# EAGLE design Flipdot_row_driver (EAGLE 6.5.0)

## Sheet 1 of 2: Flip dot driver
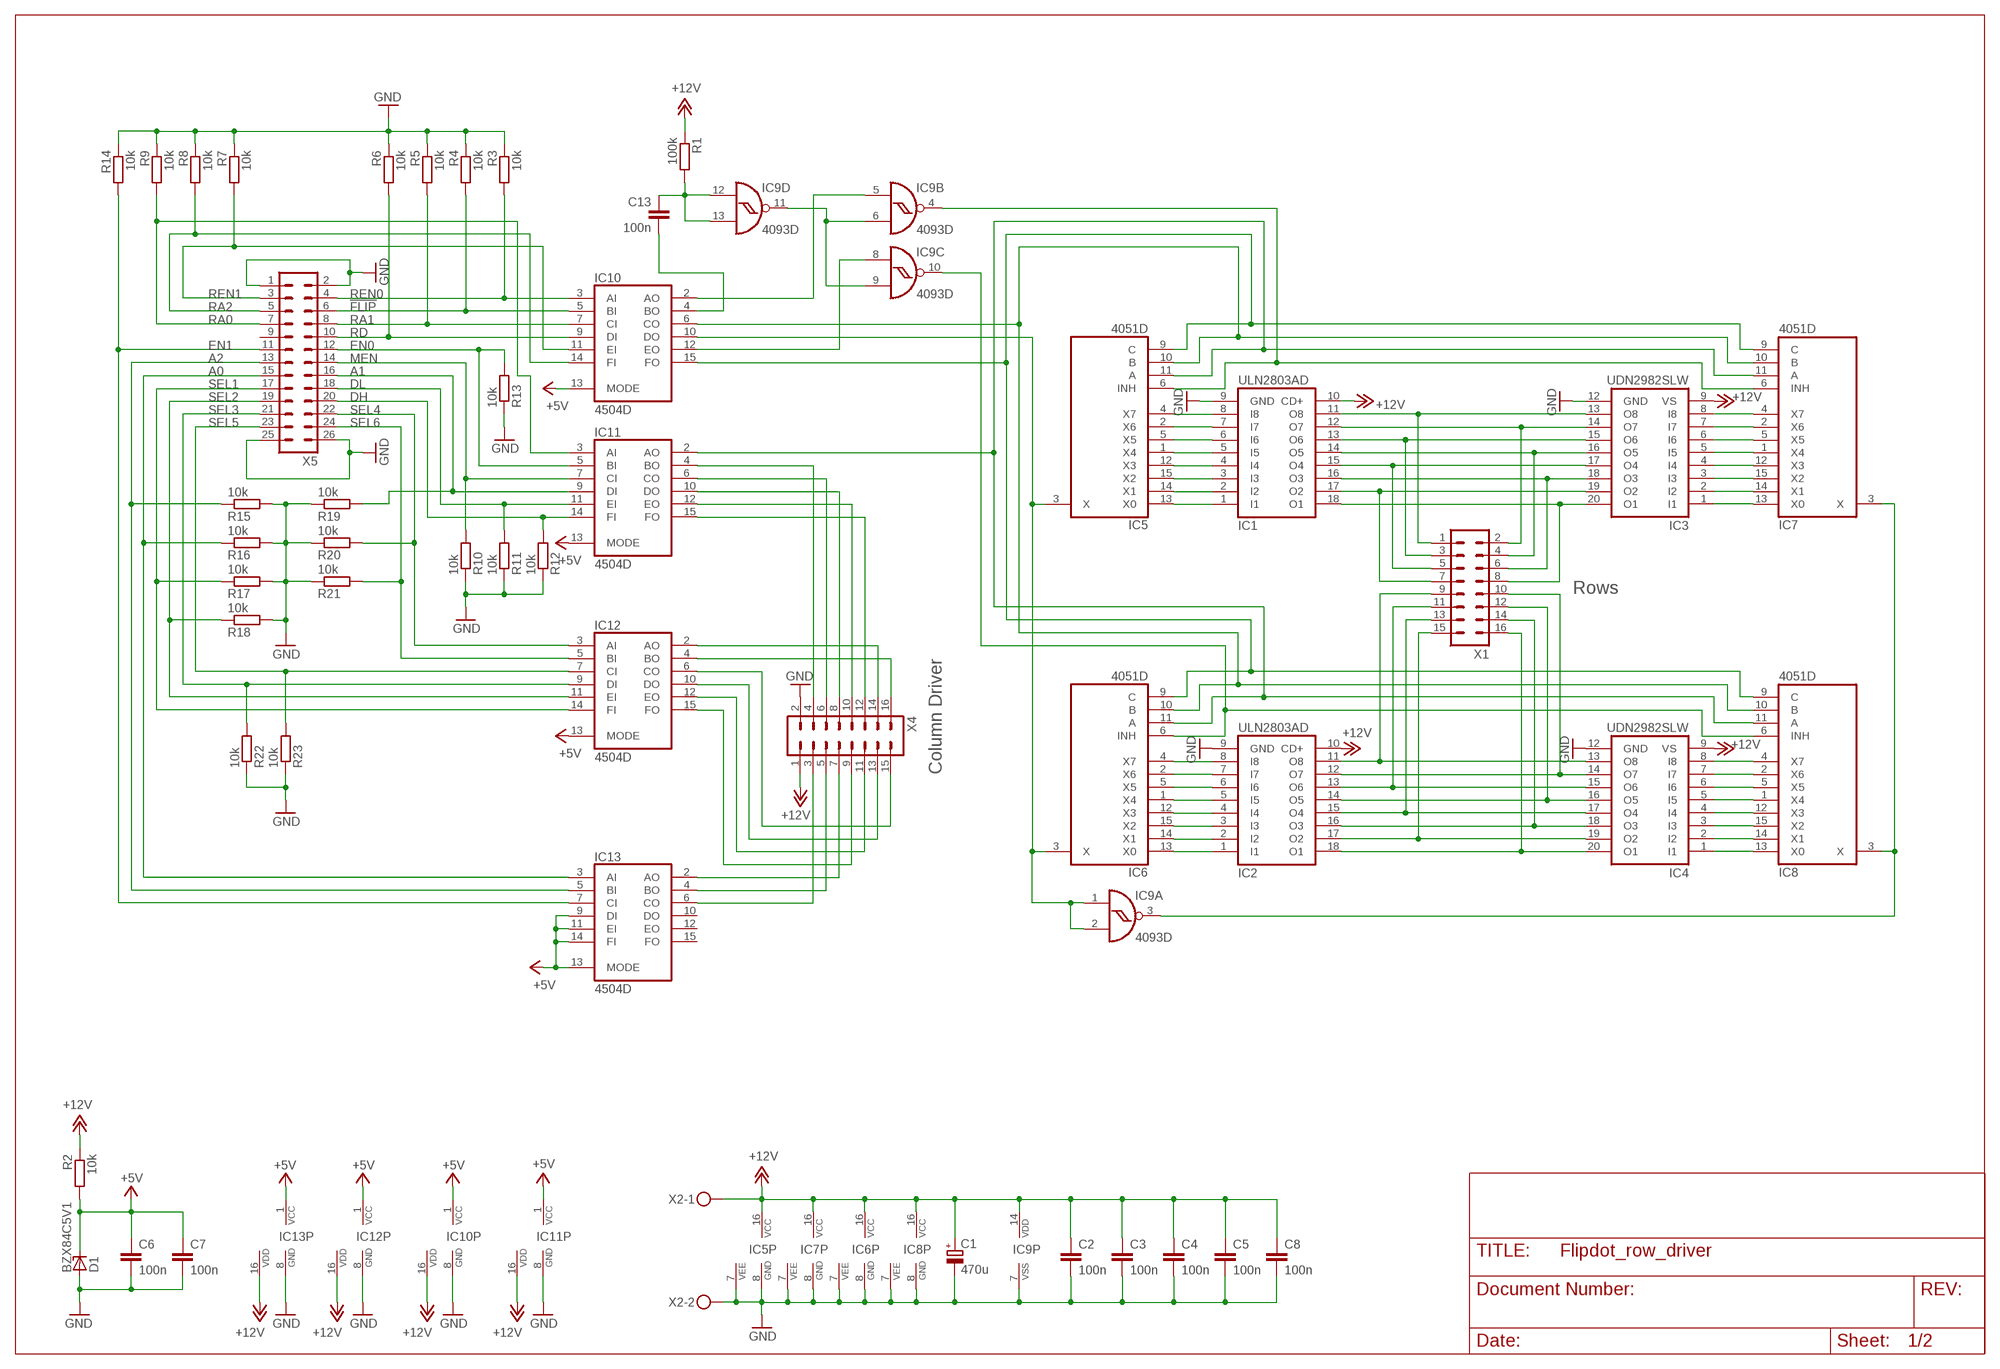
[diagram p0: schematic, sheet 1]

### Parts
C1  470u  CPOL-EUE3.5-8  [E3,5-8]
C2  100n  C-EUC0603K  [C0603K]
C3  100n  C-EUC0603K  [C0603K]
C4  100n  C-EUC0603K  [C0603K]
C5  100n  C-EUC0603K  [C0603K]
C6  100n  C-EUC0603K  [C0603K]
C7  100n  C-EUC0603K  [C0603K]
C8  100n  C-EUC0603K  [C0603K]
C13  100n  C-EUC0603K  [C0603K]
D1  BZX84C5V1  BZX84CSMD  [TO236]
IC1  ULN2803AD  [SO18W]
IC2  ULN2803AD  [SO18W]
IC3  UDN2982SLW  UDN2984SLW  [SO20W]
IC4  UDN2982SLW  UDN2984SLW  [SO20W]
IC5  4051D  [SO16]
IC6  4051D  [SO16]
IC7  4051D  [SO16]
IC8  4051D  [SO16]
IC9  4093D  [SO14]
IC10  4504D  [SO16]
IC11  4504D  [SO16]
IC12  4504D  [SO16]
IC13  4504D  [SO16]
R1  100k  R-EU_R0603  [R0603]
R2  10k  R-EU_R0603  [R0603]
R3  10k  R-EU_R0603  [R0603]
R4  10k  R-EU_R0603  [R0603]
R5  10k  R-EU_R0603  [R0603]
R6  10k  R-EU_R0603  [R0603]
R7  10k  R-EU_R0603  [R0603]
R8  10k  R-EU_R0603  [R0603]
R9  10k  R-EU_R0603  [R0603]
R10  10k  R-EU_R0603  [R0603]
R11  10k  R-EU_R0603  [R0603]
R12  10k  R-EU_R0603  [R0603]
R13  10k  R-EU_R0603  [R0603]
R14  10k  R-EU_R0603  [R0603]
R15  10k  R-EU_R0603  [R0603]
R16  10k  R-EU_R0603  [R0603]
R17  10k  R-EU_R0603  [R0603]
R18  10k  R-EU_R0603  [R0603]
R19  10k  R-EU_R0603  [R0603]
R20  10k  R-EU_R0603  [R0603]
R21  10k  R-EU_R0603  [R0603]
R22  10k  R-EU_R0603  [R0603]
R23  10k  R-EU_R0603  [R0603]
X1  ML16  [ML16]
X2  MKDSN1,5/2-5,08  [MKDSN1,5/2-5,08]
X4  ML16  [ML16]
X5  ML26  [ML26]

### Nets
!FLIP: IC10.5(BI) R4.2 X5.6
+5V: C6.1 C7.1 D1.C IC10.1(VCC) IC10.13(MODE) IC11.1(VCC) IC11.13(MODE) IC12.1(VCC) IC12.13(MODE) IC13.1(VCC) IC13.9(DI) IC13.11(EI) IC13.13(MODE) IC13.14(FI) R2.2
+12V: C1.+ C2.1 C3.1 C4.1 C5.1 C8.1 IC1.10(CD+) IC2.10(CD+) IC3.9(VS) IC4.9(VS) IC5.16(VCC) IC6.16(VCC) IC7.16(VCC) IC8.16(VCC) IC9.14(P:VDD) IC10.16(VDD) IC11.16(VDD) IC12.16(VDD) IC13.16(VDD) R1.1 R2.1 X2.1 X4.1 ; also sheet 2
A0: IC13.3(AI) R16.1 X5.15
A1: IC11.9(DI) R19.2 X5.16
A2: IC13.5(BI) R15.1 X5.13
DH: IC11.14(FI) R12.2 X5.20
DL: IC11.11(EI) R11.2 X5.18
EN0: IC11.5(BI) R13.2 X5.12
EN1: IC13.7(CI) R14.2 X5.11
GND: C1.- C2.2 C3.2 C4.2 C5.2 C6.2 C7.2 C8.2 D1.A IC1.9(GND) IC2.9(GND) IC3.12(GND) IC4.12(GND) IC5.7(VEE) IC5.8(GND) IC6.7(VEE) IC6.8(GND) IC7.7(VEE) IC7.8(GND) IC8.7(VEE) IC8.8(GND) IC9.7(P:VSS) IC10.8(GND) IC11.8(GND) IC12.8(GND) IC13.8(GND) R3.1 R4.1 R5.1 R6.1 R7.1 R8.1 R9.1 R10.1 R11.1 R12.1 R13.1 R14.1 R15.2 R16.2 R17.2 R18.2 R19.1 R20.1 R21.1 R22.1 R23.1 X2.2 X4.2 X5.1 X5.2 X5.25 X5.26 ; also sheet 2
MEN: IC11.7(CI) R10.2 X5.14
N$1: IC11.4(BO) X4.4
N$2: IC1.12(O7) IC3.14(O7) X1.2
N$3: IC11.6(CO) X4.6
N$4: IC1.14(O5) IC3.16(O5) X1.4
N$5: IC11.10(DO) X4.8
N$6: IC1.16(O3) IC3.18(O3) X1.6
N$7: IC11.12(EO) X4.10
N$8: IC1.18(O1) IC3.20(O1) X1.8
N$9: IC11.15(FO) X4.12
N$10: IC1.11(O8) IC3.13(O8) X1.1
N$11: IC12.2(AO) X4.14
N$12: IC1.13(O6) IC3.15(O6) X1.3
N$13: IC12.4(BO) X4.16
N$14: IC1.15(O4) IC3.17(O4) X1.5
N$15: IC13.6(CO) X4.3
N$16: IC1.17(O2) IC3.19(O2) X1.7
N$17: IC1.8(I8) IC5.4(X7)
N$18: IC1.7(I7) IC5.2(X6)
N$19: IC1.6(I6) IC5.5(X5)
N$20: IC1.5(I5) IC5.1(X4)
N$21: IC1.4(I4) IC5.12(X3)
N$22: IC1.3(I3) IC5.15(X2)
N$23: IC1.2(I2) IC5.14(X1)
N$24: IC1.1(I1) IC5.13(X0)
N$25: IC3.5(I5) IC7.1(X4)
N$26: IC3.7(I7) IC7.2(X6)
N$27: IC3.8(I8) IC7.4(X7)
N$28: IC3.6(I6) IC7.5(X5)
N$29: IC3.4(I4) IC7.12(X3)
N$30: IC3.1(I1) IC7.13(X0)
N$31: IC3.2(I2) IC7.14(X1)
N$32: IC3.3(I3) IC7.15(X2)
N$33: IC13.4(BO) X4.5
N$34: IC13.2(AO) X4.7
N$35: IC6.6(INH) IC8.6(INH) IC9.10(C:O)
N$36: C13.1 IC9.12(D:I0) IC9.13(D:I1) R1.2
N$37: IC12.15(FO) X4.9
N$38: IC12.12(EO) X4.11
N$39: IC9.6(B:I1) IC9.9(C:I1) IC9.11(D:O)
N$40: IC12.10(DO) X4.13
N$41: IC12.6(CO) X4.15
N$43: IC5.3(X) IC6.3(X) IC9.1(A:I0) IC9.2(A:I1) IC10.10(DO)
N$46: IC2.12(O7) IC4.14(O7) X1.10
N$48: IC2.14(O5) IC4.16(O5) X1.12
N$50: IC2.16(O3) IC4.18(O3) X1.14
N$52: IC2.18(O1) IC4.20(O1) X1.16
N$54: IC2.11(O8) IC4.13(O8) X1.9
N$56: IC2.13(O6) IC4.15(O6) X1.11
N$58: IC2.15(O4) IC4.17(O4) X1.13
N$60: IC2.17(O2) IC4.19(O2) X1.15
N$61: IC2.8(I8) IC6.4(X7)
N$62: IC2.7(I7) IC6.2(X6)
N$63: IC2.6(I6) IC6.5(X5)
N$64: IC2.5(I5) IC6.1(X4)
N$65: IC2.4(I4) IC6.12(X3)
N$66: IC2.3(I3) IC6.15(X2)
N$67: IC2.2(I2) IC6.14(X1)
N$68: IC2.1(I1) IC6.13(X0)
N$69: IC4.5(I5) IC8.1(X4)
N$70: IC4.7(I7) IC8.2(X6)
N$71: IC4.8(I8) IC8.4(X7)
N$72: IC4.6(I6) IC8.5(X5)
N$73: IC4.4(I4) IC8.12(X3)
N$74: IC4.1(I1) IC8.13(X0)
N$75: IC4.2(I2) IC8.14(X1)
N$76: IC4.3(I3) IC8.15(X2)
N$77: IC5.6(INH) IC7.6(INH) IC9.4(B:O)
N$100: IC9.5(B:I0) IC10.2(AO)
N$101: C13.2 IC10.4(BO)
N$102: IC5.10(B) IC6.10(B) IC7.10(B) IC8.10(B) IC10.6(CO)
N$104: IC9.8(C:I0) IC10.12(EO)
N$105: IC5.9(C) IC6.9(C) IC7.9(C) IC8.9(C) IC10.15(FO)
N$106: IC5.11(A) IC6.11(A) IC7.11(A) IC8.11(A) IC11.2(AO)
N$110: IC7.3(X) IC8.3(X) IC9.3(A:O)
RA0: IC11.3(AI) R9.2 X5.7
RA1: IC10.7(CI) R5.2 X5.8
RA2: IC10.14(FI) R8.2 X5.5
RD: IC10.9(DI) R6.2 X5.10
REN0: IC10.3(AI) R3.2 X5.4
REN1: IC10.11(EI) R7.2 X5.3
SEL1: IC12.14(FI) R17.1 X5.17
SEL2: IC12.11(EI) R18.1 X5.19
SEL3: IC12.9(DI) R22.2 X5.21
SEL4: IC12.3(AI) R20.2 X5.22
SEL5: IC12.7(CI) R23.2 X5.23
SEL6: IC12.5(BI) R21.2 X5.24
Unconnected: IC13.10(DO) IC13.12(EO) IC13.15(FO) X5.9

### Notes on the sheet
- Rows
- Column Driver

## Sheet 2 of 2: Flip dot master
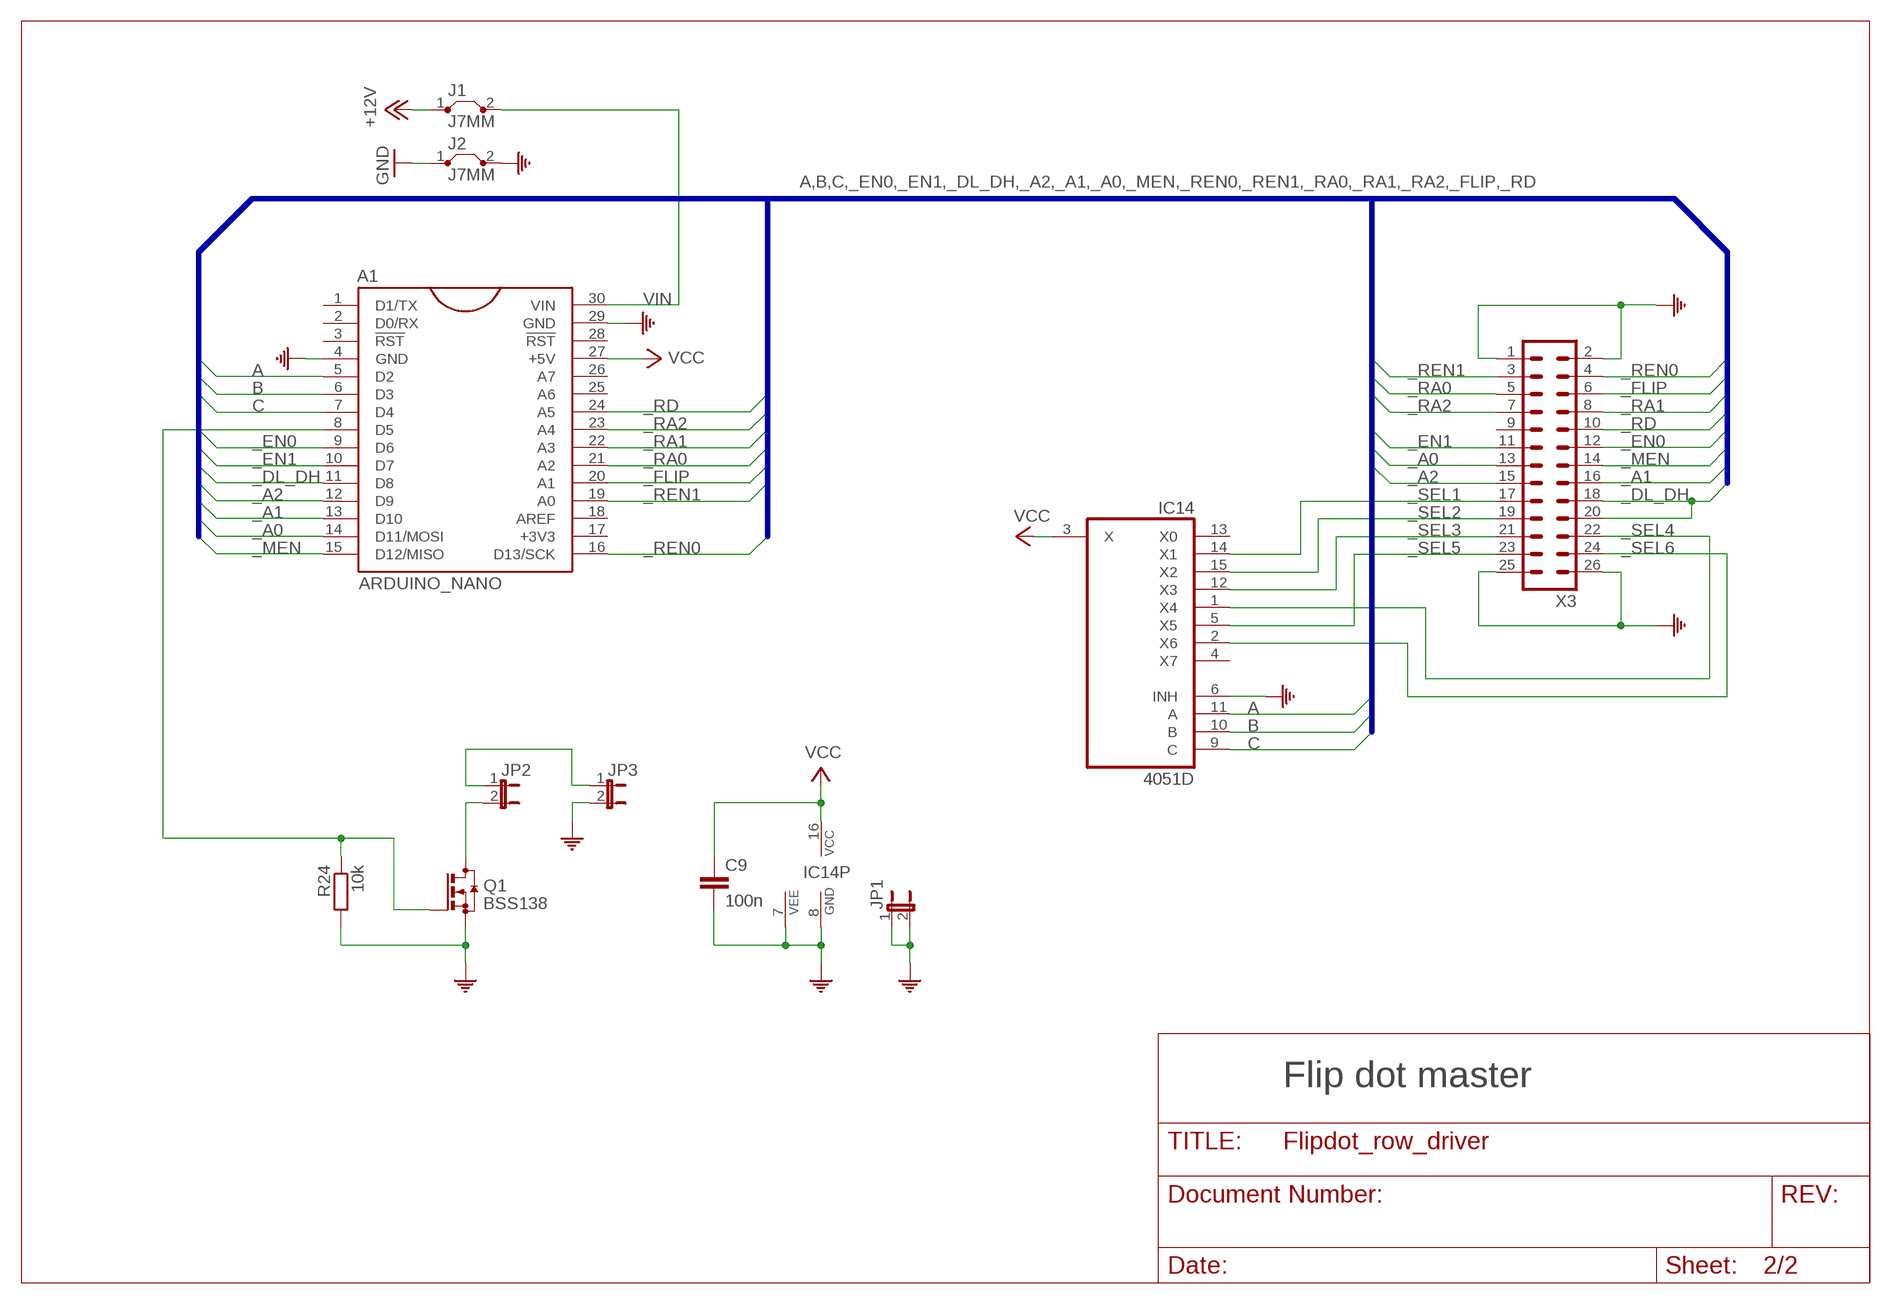
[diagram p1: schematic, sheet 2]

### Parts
A1  ARDUINO_NANO  [ARDUINO_NANO]
C9  100n  C-EUC0603K  [C0603K]
IC14  4051D  [SO16]
J1  J7MM  [07]
J2  J7MM  [07]
JP1  JP1E  [JP1]
JP2  JP1E  [JP1]
JP3  JP1E  [JP1]
Q1  BSS138  BSS123  [SOT23]
R24  10k  R-EU_R0603  [R0603]
X3  ML26  [ML26]

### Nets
+12V: J1.1 ; also sheet 1
_A0: A1.14(D11/MOSI) X3.13
_A1: A1.13(D10) X3.16
_A2: A1.12(D9) X3.15
_DL_DH: A1.11(D8) X3.18 X3.20
_EN0: A1.9(D6) X3.12
_EN1: A1.10(D7) X3.11
_FLIP: A1.20(A1) X3.6
_MEN: A1.15(D12/MISO) X3.14
_RA0: A1.21(A2) X3.5
_RA1: A1.22(A3) X3.8
_RA2: A1.23(A4) X3.7
_RD: A1.24(A5) X3.10
_REN0: A1.16(D13/SCK) X3.4
_REN1: A1.19(A0) X3.3
_SEL1: IC14.14(X1) X3.17
_SEL2: IC14.15(X2) X3.19
_SEL3: IC14.12(X3) X3.21
_SEL4: IC14.1(X4) X3.22
_SEL5: IC14.5(X5) X3.23
_SEL6: IC14.2(X6) X3.24
A: A1.5(D2) IC14.11(A)
B: A1.6(D3) IC14.10(B)
C: A1.7(D4) IC14.9(C)
COM: A1.4(GND) A1.29(GND) C9.2 IC14.6(INH) IC14.7(VEE) IC14.8(GND) J2.2 JP1.1 JP1.2 JP3.2 Q1.2(S) R24.2 X3.1 X3.2 X3.25 X3.26
GND: J2.1 ; also sheet 1
N$42: A1.8(D5) Q1.1(G) R24.1
N$44: JP2.2 Q1.3(D)
N$45: JP2.1 JP3.1
VCC: A1.27(+5V) C9.1 IC14.3(X) IC14.16(VCC)
VIN: A1.30(VIN) J1.2
Unconnected: A1.1(D1/TX) A1.2(D0/RX) A1.3(!RST) A1.17(+3V3) A1.18(AREF) A1.25(A6) A1.26(A7) A1.28(!RST) IC14.4(X7) IC14.13(X0) X3.9

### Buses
A,B,C,_EN0,_EN1,_DL_DH,_A2,_A1,_A0,_MEN,_REN0,_REN1,_RA0,_RA1,_RA2,_FLIP,_RD

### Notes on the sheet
- Flip dot master

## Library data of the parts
A1 = Brunner:ARDUINO_NANO: Arduino Nano plug in module
C1 = rcl:CPOL-EU: POLARIZED CAPACITOR, European symbol
C2-C9 C13 = rcl:C-EU: CAPACITOR, European symbol
D1 = diode:BZX84CSMD: Z DIODE
IC1 IC2 = Brunner:ULN2803A: DRIVER ARRAY
IC3 IC4 = uln-udn:UDN298*: DRIVER ARRAY Source: Allegro Microsystems Inc. / UDN2981-UDN2984.pdf
IC5-IC8 IC14 = 40xx:4051: 8-channel ANALOG MULTIPLEXER
IC9 = 40xx:4093: Quad 2-input NAND schmitt trigger
IC10-IC13 = 45xx:4504: TTL or CMOS to CMOS hex LEVEL SHIFTER
J1 J2 = jumper:J: Bridge
JP1-JP3 = jumper:JP1E: JUMPER
Q1 = transistor-small-signal:BSS123: N-CHANNEL MOS FET
R1-R24 = rcl:R-EU_: RESISTOR, European symbol
X1 X4 = con-ml:ML16: HARTING; OC_FARNELL: unknown; OC_NEWARK: unknown
X2 = con-phoenix-508:MKDSN1,5/2-5,08: MKDSN 1,5/ 2-5,08 Printklemme; MPN: MKDSN 1,5/2-5.08; OC_FARNELL: 1792903; OC_NEWARK: 30M2397
X3 X5 = con-ml:ML26: HARTING; OC_FARNELL: unknown; OC_NEWARK: unknown

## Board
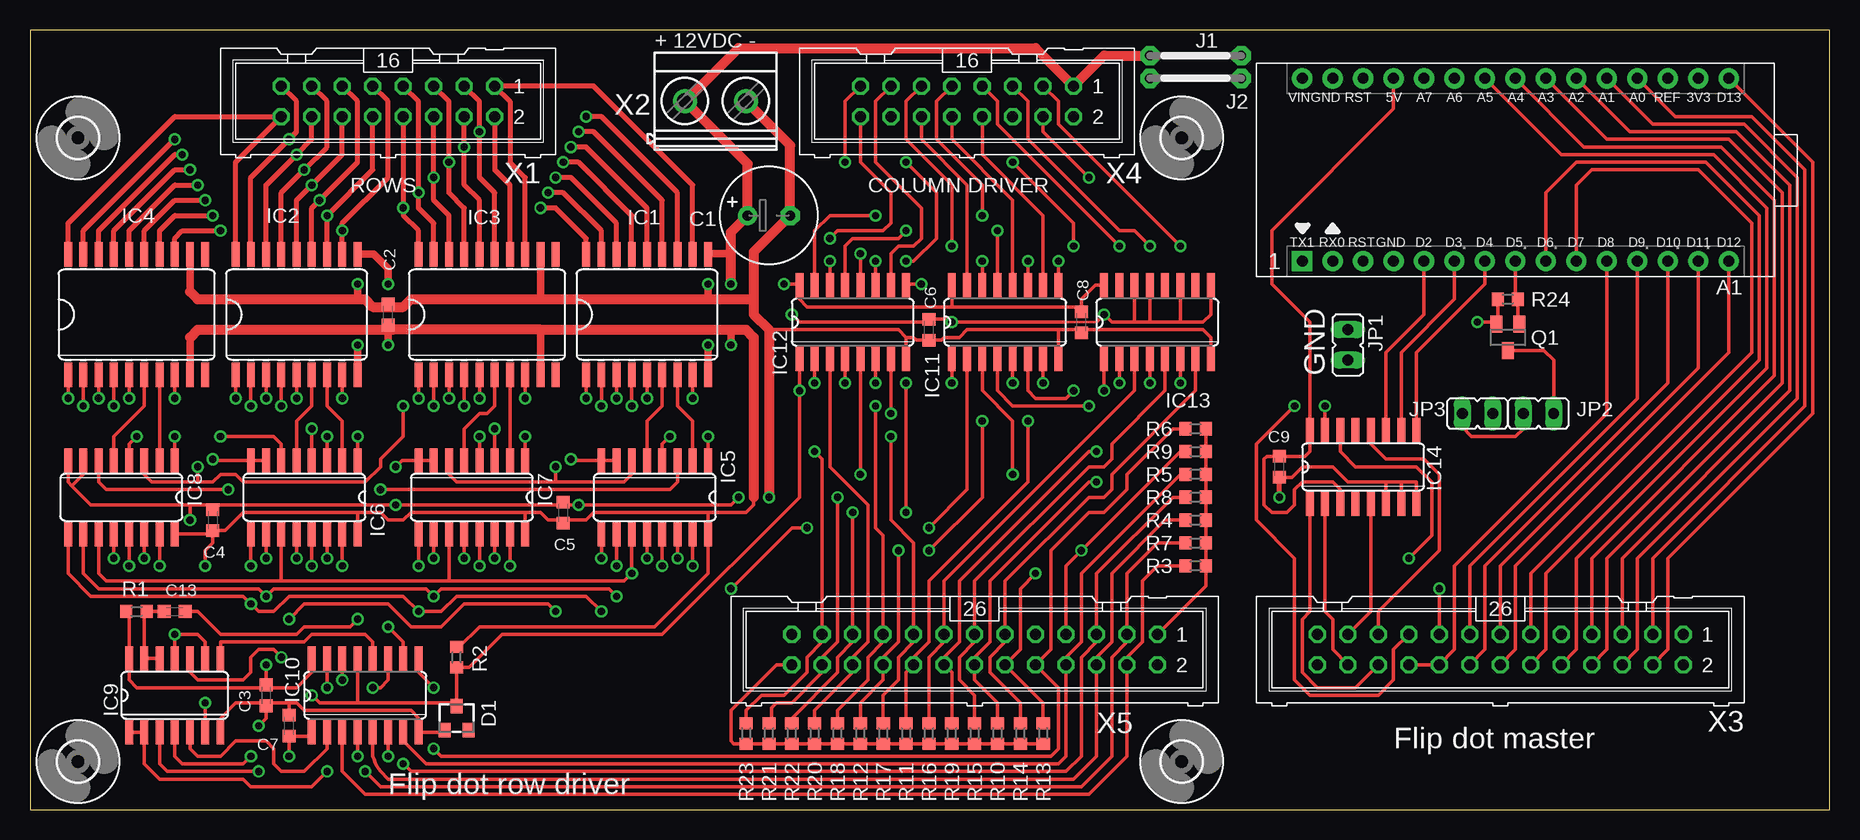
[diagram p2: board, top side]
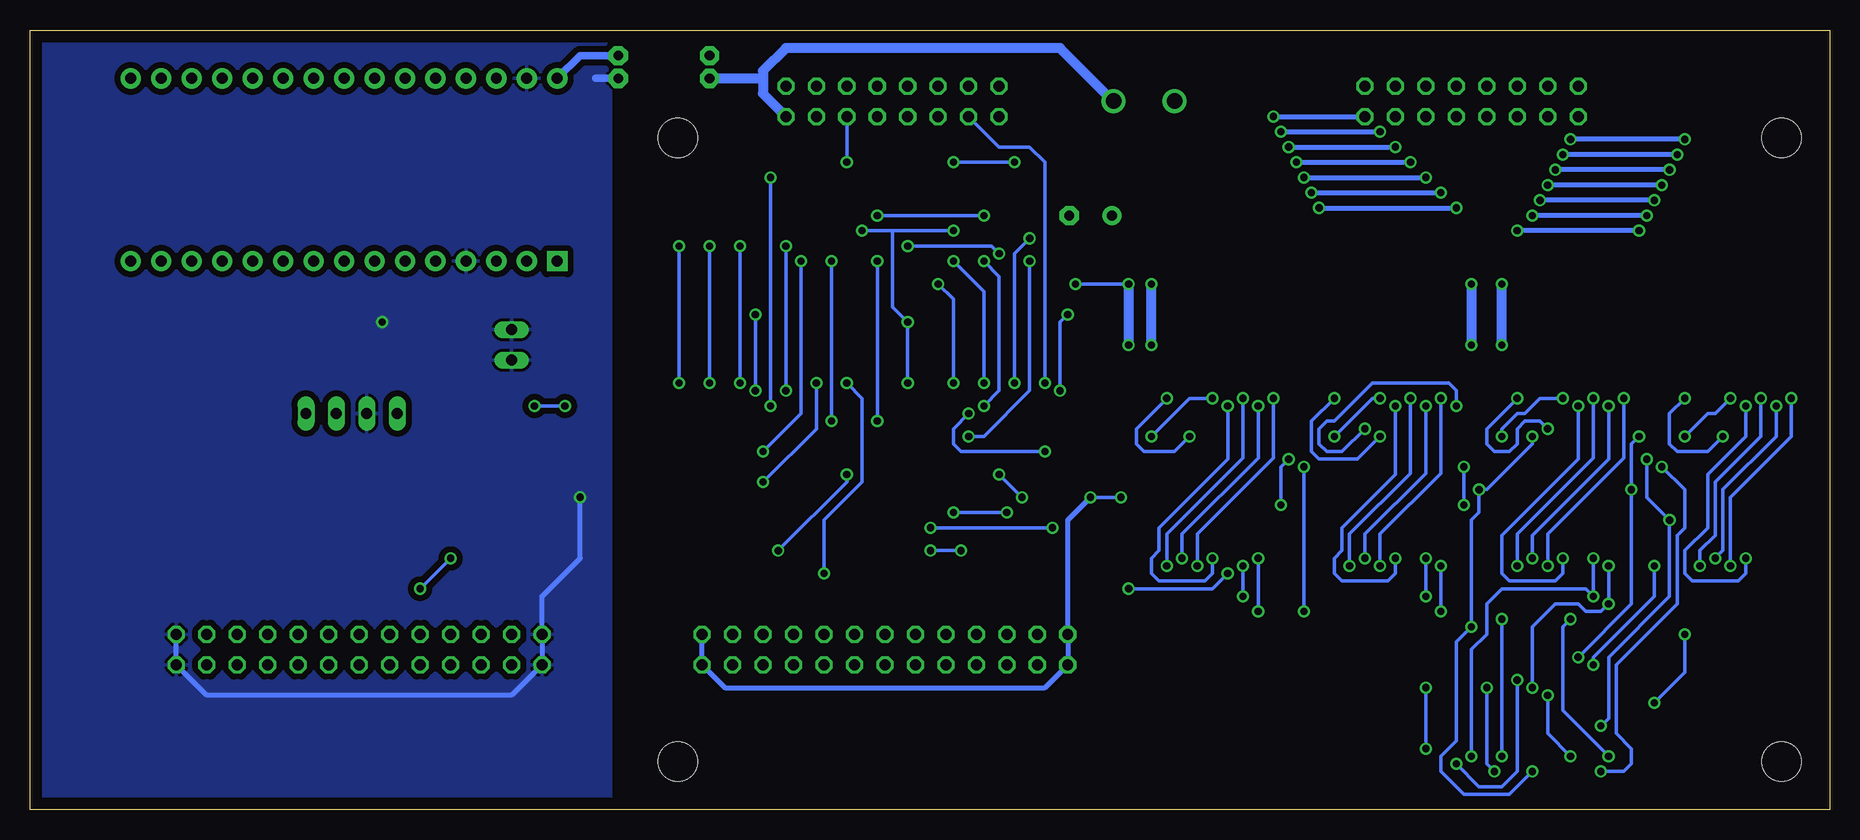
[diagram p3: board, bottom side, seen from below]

Size 150 x 65 mm. Coordinates in mm from the lower left corner, seen from the top.
Outline: 0,0 150,0 150,65 0,65 0,0
Copper layers (1*16): Top 0.035mm / dielectric 1.5mm / Bottom 0.035mm
Design rules "default *": minimum track width 0.3mm, minimum drill 0.5mm, track to track 0.3mm, track to pad 0.3mm, pad to pad 0.3mm, via to via 0.3mm, smd to smd 8mil, copper to edge 1mm, drill to drill 8mil, minimum pad ring 10mil, minimum via ring 8mil, stop-mask expansion 4mil, vias tented up to drill 0mil, thermal gap 10mil

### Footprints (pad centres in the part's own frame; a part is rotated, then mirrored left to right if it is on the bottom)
ARDUINO_NANO = drill 0.914 pad 1.676 square: 1 17.78,7.62 | drill 0.914 pad 1.676: 2 15.24,7.62; 3 12.7,7.62; 4 10.16,7.62; 5 7.62,7.62; 6 5.08,7.62; 7 2.54,7.62; 8 0,7.62; 9 -2.54,7.62; 10 -5.08,7.62; 11 -7.62,7.62; 12 -10.16,7.62; 13 -12.7,7.62; 14 -15.24,7.62; 15 -17.78,7.62; 16 -17.78,-7.62; 17 -15.24,-7.62; 18 -12.7,-7.62; 19 -10.16,-7.62; 20 -7.62,-7.62; 21 -5.08,-7.62; 22 -2.54,-7.62; 23 0,-7.62; 24 2.54,-7.62; 25 5.08,-7.62; 26 7.62,-7.62; 27 10.16,-7.62; 28 12.7,-7.62; 29 15.24,-7.62; 30 17.78,-7.62
E3,5-8 = drill 0.813 pad 1.6: + -1.778,0 | drill 0.813 pad 1.6 octagon: - 1.778,0
C0603K = smd 1.05 x 1.08: 1 -0.875,0; 2 0.875,0
TO236 = smd 1 x 1.2: A -1,-1; C 0,1; NC 1,-1
SO18W = smd 0.66 x 2.032: 1 -5.08,-5.029; 2 -3.81,-5.029; 3 -2.54,-5.029; 4 -1.27,-5.029; 5 0,-5.029; 6 1.27,-5.029; 7 2.54,-5.029; 8 3.81,-5.029; 9 5.08,-5.029; 10 5.08,5.029; 11 3.81,5.029; 12 2.54,5.029; 13 1.27,5.029; 14 0,5.029; 15 -1.27,5.029; 16 -2.54,5.029; 17 -3.81,5.029; 18 -5.08,5.029
SO20W = smd 0.66 x 2.032: 1 -5.715,-5.029; 2 -4.445,-5.029; 3 -3.175,-5.029; 4 -1.905,-5.029; 5 -0.635,-5.029; 6 0.635,-5.029; 7 1.905,-5.029; 8 3.175,-5.029; 9 4.445,-5.029; 10 5.715,-5.029; 11 5.715,5.029; 12 4.445,5.029; 13 3.175,5.029; 14 1.905,5.029; 15 0.635,5.029; 16 -0.635,5.029; 17 -1.905,5.029; 18 -3.175,5.029; 19 -4.445,5.029; 20 -5.715,5.029
SO16 = smd 0.66 x 2.032: 1 -4.445,-3.073; 2 -3.175,-3.073; 3 -1.905,-3.073; 4 -0.635,-3.073; 5 0.635,-3.073; 6 1.905,-3.073; 7 3.175,-3.073; 8 4.445,-3.073; 9 4.445,3.073; 10 3.175,3.073; 11 1.905,3.073; 12 0.635,3.073; 13 -0.635,3.073; 14 -1.905,3.073; 15 -3.175,3.073; 16 -4.445,3.073
SO14 = smd 0.66 x 2.032: 1 -3.81,-3.073; 2 -2.54,-3.073; 3 -1.27,-3.073; 4 0,-3.073; 5 1.27,-3.073; 6 2.54,-3.073; 7 3.81,-3.073; 8 3.81,3.073; 9 2.54,3.073; 10 1.27,3.073; 11 0,3.073; 12 -1.27,3.073; 13 -2.54,3.073; 14 -3.81,3.073
07 = drill 0.813 pad 1.6 octagon: 1 -3.81,0; 2 3.81,0
JP1 = drill 0.914 long: 1 0,-1.27; 2 0,1.27
SOT23 = smd 1 x 1.4: 1 -0.95,-1.1; 2 0.95,-1.1; 3 0,1.1
R0603 = smd 1 x 1.1: 1 -0.85,0; 2 0.85,0
3,3 = hole 3.3: 0,0
ML16 = drill 0.914 octagon: 1 -8.89,-1.27; 2 -8.89,1.27; 3 -6.35,-1.27; 4 -6.35,1.27; 5 -3.81,-1.27; 6 -3.81,1.27; 7 -1.27,-1.27; 8 -1.27,1.27; 9 1.27,-1.27; 10 1.27,1.27; 11 3.81,-1.27; 12 3.81,1.27; 13 6.35,-1.27; 14 6.35,1.27; 15 8.89,-1.27; 16 8.89,1.27
MKDSN1,5/2-5,08 = drill 1.3 pad 2: 1 -2.561,0.025; 2 2.519,0.025
ML26 = drill 0.914 octagon: 1 -15.24,-1.27; 2 -15.24,1.27; 3 -12.7,-1.27; 4 -12.7,1.27; 5 -10.16,-1.27; 6 -10.16,1.27; 7 -7.62,-1.27; 8 -7.62,1.27; 9 -5.08,-1.27; 10 -5.08,1.27; 11 -2.54,-1.27; 12 -2.54,1.27; 13 0,-1.27; 14 0,1.27; 15 2.54,-1.27; 16 2.54,1.27; 17 5.08,-1.27; 18 5.08,1.27; 19 7.62,-1.27; 20 7.62,1.27; 21 10.16,-1.27; 22 10.16,1.27; 23 12.7,-1.27; 24 12.7,1.27; 25 15.24,-1.27; 26 15.24,1.27

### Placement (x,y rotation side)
A1  123.83,53.34 180 top
C1  61.59,49.53 0 top
C2  29.84,41.27 90 top
C3  19.68,9.53 270 top
C4  15.24,24.13 90 top
C5  44.45,24.77 90 top
C6  74.93,40.01 270 top
C7  21.59,6.99 90 top
C8  87.63,40.64 270 top
C9  104.14,28.57 270 top
C13  12.06,16.51 0 top
D1  35.56,7.62 0 top
IC1  51.44,41.27 0 top
IC2  22.23,41.27 0 top
IC3  38.1,41.27 0 top
IC4  8.89,41.27 0 top
IC5  52.07,26.04 180 top
IC6  22.86,26.04 180 top
IC7  36.83,26.04 180 top
IC8  7.62,26.04 180 top
IC9  12.06,9.53 0 top
IC10  27.94,9.53 0 top
IC11  81.28,40.64 0 top
IC12  68.58,40.64 0 top
IC13  93.98,40.64 0 top
IC14  111.12,28.57 0 top
J1  97.16,62.87 0 top
J2  97.16,60.96 0 top
JP1  109.86,38.73 180 top
JP2  125.73,33.02 270 top
JP3  120.65,33.02 270 top
Q1  123.19,39.37 180 top
R1  8.89,16.51 0 top
R2  35.56,12.7 270 top
R3  97.16,20.32 180 top
R4  97.16,24.13 180 top
R5  97.16,27.94 180 top
R6  97.16,31.75 180 top
R7  97.16,22.23 180 top
R8  97.16,26.04 180 top
R9  97.16,29.84 180 top
R10  80.64,6.35 90 top
R11  73.03,6.35 90 top
R12  69.22,6.35 90 top
R13  84.45,6.35 90 top
R14  82.55,6.35 90 top
R15  78.74,6.35 270 top
R16  74.93,6.35 270 top
R17  71.12,6.35 270 top
R18  67.31,6.35 270 top
R19  76.83,6.35 90 top
R20  65.41,6.35 90 top
R21  61.59,6.35 90 top
R22  63.5,6.35 90 top
R23  59.69,6.35 90 top
R24  123.19,42.55 180 top
U$1  [3,3]  4,56 0 top
U$2  [3,3]  96,4 0 top
U$3  [3,3]  4,4 0 top
U$4  [3,3]  96,56 0 top
U$8  [A4L-LOC]  not placed on the board
X1  29.84,59.05 180 top
X2  57.15,59.05 0 top
X3  122.56,13.34 180 top
X4  78.11,59.05 180 top
X5  78.74,13.34 180 top

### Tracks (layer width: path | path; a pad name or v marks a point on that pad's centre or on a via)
!FLIP
  Top 0.305: IC10.5 28.57,4.45 arc18 29.21,3.17 29.84,2.54 87,2.54 88.9,4.45 X5.6 88.9,12.7 90.17,13.97 90.17,19.68 94.61,24.13 R4.2
+5V  (via drill 0.6)
  Top 0.2: 88.9,40.64 86.36,40.64
  Top 0.305: IC10.1 23.15,6.11 C7.1 v21.59,4.45 | IC10.13 27.3,8.89 | 27.3,8.89 35.29,8.89 D1.C R2.2 36.62,11.85 39.37,14.61 52.7,14.61 64.14,26.04 v64.14,34.92 IC12.1 | 27.3,8.89 24.13,8.89 v23.5,9.53 | 92.08,40.64 93.34,40.64 | 93.34,40.64 95.89,40.64 | 95.89,40.64 97.79,40.64 98.42,41.27 IC13.9 | IC13.14 92.08,40.64 | IC13.13 93.34,40.64 | IC13.11 95.89,40.64 | IC13.1 v89.53,34.92 | IC11.1 v76.83,35.56 | v63.5,41.27 64.14,40.64 74.69,40.64 C6.1 76.59,40.88 v76.83,40.64 86.36,40.64 | IC11.13 v80.64,48.26 | IC12.13 67.94,46.99 68.58,47.62 72.39,47.62 v73.03,48.26 | 92.08,40.64 90.17,40.64 v89.53,41.27 88.9,40.64
  Bottom 0.305: v23.5,9.53 23.5,6.35 v21.59,4.45 | v89.53,34.92 v89.53,41.27 | v76.83,35.56 v76.83,40.64 78.11,41.91 78.11,48.26 | v64.14,34.92 64.14,40.64 v63.5,41.27 | v80.64,48.26 78.11,48.26 | v73.03,48.26 78.11,48.26
+12V  (via drill 0.6)
  Top 0.305: IC8.16 14.95,22.96 C4.1 | C4.1 16.27,23.25 17.78,24.77 27.3,24.77 | 27.3,24.77 IC6.16 | 27.3,24.77 29.21,24.77 29.84,24.13 31.11,24.13 31.75,24.77 41.27,24.77 | 41.27,24.77 IC7.16 41.27,22.86 | 56.52,24.77 46.99,24.77 46.35,24.13 44.69,24.13 C5.1 44.21,24.13 43.18,24.13 42.55,24.77 41.27,24.77 | 56.52,24.77 IC5.16 56.52,19.68 52.07,15.24 37.47,15.24 35.77,13.55 R2.1 | 56.52,24.77 59.69,24.77 60.33,25.4 60.33,26.04 | IC10.16 23.5,11.43 22.23,10.16 19.93,10.16 C3.1 | C3.1 19.45,10.16 8.89,10.16 8.26,10.79 IC9.14 8.26,16.3 R1.1 | C4.1 15.24,22.23 14.61,21.59 v14.61,20.32 | v19.68,12.06 C3.1 | v62.87,43.81 64.03,43.81 IC12.16 64.14,42.55 64.77,41.91 76.83,41.91 | 76.83,41.91 87.23,41.91 C8.1 87.63,42.55 88.8,43.71 IC13.16 | IC11.16 76.83,41.91
  Top 0.61: IC4.9 13.34,39.37 | IC3.9 42.55,40.01 | IC2.10 28.63,46.3 29.84,45.09 v29.84,43.81 | v29.84,38.73 C2.1 30.24,40.01 | v58.42,38.73 58.42,40.01 | IC1.10 56.57,46.35 58.42,46.35
  Top 0.813: 13.34,39.37 13.97,40.01 30.24,40.01 42.55,40.01 58.42,40.01 59.69,40.01 60.33,39.37 60.33,26.04 | v58.42,43.81 58.42,46.35 58.42,48.13 C1.+ 59.82,53.85 X2.1 | 54.61,59.06 X2.1 | X2.1 54.63,59.08 59.05,63.5 83.82,63.5 X4.1 89.53,62.87 J1.1
  Bottom 0.305: v14.61,20.32 14.61,17.78 19.68,12.7 v19.68,12.06 | v58.42,43.81 v62.87,43.81
  Bottom 0.813: v29.84,43.81 v29.84,38.73 | v58.42,43.81 v58.42,38.73
_A0
  Top 0.305: X3.13 122.56,20.32 139.06,36.83 A1.14
_A1
  Top 0.305: X3.16 121.28,13.34 121.28,20.32 136.53,35.56 A1.13
_A2
  Top 0.305: X3.15 120.02,20.32 133.99,34.29 A1.12
_DL_DH
  Top 0.305: A1.11 131.44,33.02 118.75,20.32 118.75,13.34 X3.18 X3.20
_EN0
  Top 0.305: X3.12 126.36,13.34 126.36,19.68 144.15,37.47 144.15,49.53 139.7,53.98 128.91,53.98 126.36,51.44 A1.9
_EN1
  Top 0.305: X3.11 125.09,19.68 143.51,38.1 143.51,48.9 139.06,53.34 130.18,53.34 128.91,52.07 A1.10
_FLIP
  Top 0.305: X3.6 133.99,13.34 133.99,20.95 147.32,34.29 147.32,52.7 142.88,57.15 135.25,57.15 A1.20
_MEN
  Top 0.305: X3.14 123.83,13.34 123.83,20.32 141.6,38.1 A1.15
_RA0
  Top 0.305: A1.21 133.35,56.52 142.24,56.52 146.69,52.07 146.69,34.92 132.72,20.95 X3.5
_RA1
  Top 0.305: X3.8 131.44,13.34 131.44,20.95 146.05,35.56 146.05,51.44 141.6,55.88 131.44,55.88 A1.22
_RA2
  Top 0.305: X3.7 130.18,20.95 145.41,36.2 145.41,50.8 140.97,55.24 129.54,55.24 A1.23
_RD
  Top 0.305: X3.10 128.91,13.34 128.91,20.95 144.78,36.83 144.78,50.16 140.34,54.61 127.64,54.61 A1.24
_REN0
  Top 0.305: X3.4 136.53,13.34 136.53,20.95 148.59,33.02 148.59,53.98 A1.16
_REN1
  Top 0.305: A1.19 137.16,57.78 143.51,57.78 147.96,53.34 147.96,33.66 135.25,20.95 X3.3
_SEL1  (via drill 0.6)
  Top 0.305: IC14.14 109.22,29.84 110.49,28.57 115.57,28.57 116.84,27.3 116.84,22.86 v114.94,20.95 | v117.47,18.41 X3.17
  Bottom 0.305: v114.94,20.95 v117.47,18.41
_SEL2  (via drill 0.6)
  Top 0.305: v107.95,33.66 IC14.15 | X3.19 113.67,13.34 113.67,10.79 112.39,9.53 106.68,9.53 105.41,10.79 105.41,20.95 102.23,24.13 102.23,30.48 v105.41,33.66
  Bottom 0.305: v105.41,33.66 v107.95,33.66
_SEL3
  Top 0.305: X3.21 112.39,16.51 117.47,21.59 117.47,27.94 116.2,29.21 113.03,29.21 111.76,30.48 IC14.12
_SEL4
  Top 0.305: X3.22 110.49,10.16 107.31,10.16 106.05,11.43 106.05,15.88 106.68,16.51 IC14.1
_SEL5
  Top 0.305: X3.23 111.76,16.51 IC14.5
_SEL6
  Top 0.305: X3.24 108.58,13.34 108.58,15.88 107.95,16.51 IC14.2
A
  Top 0.305: IC14.11 113.03,38.1 116.2,41.27 A1.5
A0
  Top 0.305: IC13.3 92.08,34.92 76.2,19.05 X5.15 76.2,13.97 74.93,12.7 R16.1
A1  (via drill 0.6)
  Top 0.305: IC11.9 v85.72,45.72 | v88.9,29.84 88.27,29.84 77.47,19.05 77.47,13.97 76.2,12.7 X5.16 76.83,11.43 R19.2
  Bottom 0.305: v85.72,45.72 85.72,33.02 v88.9,29.84
A2
  Top 0.305: IC13.5 94.61,34.92 90.17,30.48 90.17,29.21 89.53,28.57 88.27,28.57 78.74,19.05 X5.13 78.74,13.97 77.47,12.7 77.47,10.79 78.74,9.53 R15.1
B
  Top 0.305: IC14.10 114.3,38.1 118.75,42.55 A1.6
C
  Top 0.305: IC14.9 115.57,38.1 121.28,43.81 A1.7
COM  (via drill 0.6)
  Top 0.305: IC14.8 115.57,27.3 114.3,27.3 | 114.3,27.3 113.03,27.3 | 113.03,27.3 109.86,27.3 108.58,28.57 106.05,28.57 105.17,27.7 C9.2 | IC14.6 113.03,27.3 | IC14.7 114.3,27.3 | R24.2 122.34,40.57 Q1.2 122.09,40.47 121.92,40.64 v120.65,40.64
  Top 0.406: v104.14,26.04 C9.2
  Bottom 0.406: X3.1 X3.2 135.25,9.53 109.86,9.53 X3.26 X3.25 107.31,17.78 104.14,20.95 v104.14,26.04
  Bottom 0.61: J2.2 102.87,60.96
  pour Bottom (isolate 0.5): 101.6,64.77 149.86,64.77 149.86,0 101.6,0
DH  (via drill 0.6)
  Top 0.305: v72.39,21.59 72.39,13.97 71.12,12.7 X5.20 71.12,10.79 69.22,8.89 R12.2 | IC11.14 v79.38,45.72 | v79.38,32.38 79.38,26.04 v74.93,21.59
  Bottom 0.305: v79.38,45.72 v79.38,32.38 | v74.93,21.59 v72.39,21.59
DL  (via drill 0.6)
  Top 0.305: IC11.11 v83.19,45.72 | v83.19,32.38 83.19,27.3 74.93,19.05 74.93,13.97 73.66,12.7 X5.18 73.03,11.43 R11.2
  Bottom 0.305: v83.19,45.72 v83.19,32.38
EN0  (via drill 0.6)
  Top 0.305: v83.82,19.68 82.55,18.41 82.55,13.34 X5.12 84.45,8.89 R13.2 | v81.92,35.56 IC11.5
  Bottom 0.305: v83.82,19.68 83.82,23.5 83.82,24.13 80.64,27.3 80.64,34.29 v81.92,35.56
EN1
  Top 0.305: IC13.7 97.16,34.92 90.17,27.94 90.17,26.67 89.53,26.04 88.27,26.04 81.28,19.05 X5.11 81.28,13.97 80.01,12.7 80.01,11.43 82.55,8.89 R14.2
GND  (via drill 0.6)
  Top 0.305: IC8.8 3.17,27.3 3.49,26.99 | 3.49,26.99 5.08,25.4 13.34,25.4 | IC8.7 4.45,27.94 3.49,26.99 | C4.2 15.24,25.4 | 15.24,25.4 13.34,25.4 | 15.24,25.4 v30.48,25.4 44.21,25.4 C5.2 44.69,25.4 v45.72,25.4 58.42,25.4 v59.05,26.04 | IC6.7 IC6.8 15.34,29.11 v15.24,29.21 | v13.34,24.13 13.34,25.4 | IC7.7 IC7.8 31.01,29.11 v30.48,28.57 | v45.09,29.21 45.19,29.11 IC5.8 IC5.7 | IC9.7 15.88,7.62 17.14,8.89 19.45,8.89 C3.2 | C3.2 19.68,8.89 21.59,8.89 | 21.59,8.89 22.23,8.89 22.86,8.26 31.75,8.26 32.38,7.62 IC10.8 34.39,6.45 D1.A | C7.2 21.59,8.89 | v19.05,6.99 19.68,7.62 C3.2 | IC12.8 73.03,39.37 | 73.03,39.37 72.39,40.01 61.59,40.01 | 85.72,40.01 78.11,40.01 77.47,39.37 76.2,39.37 75.96,39.13 C6.2 73.9,39.13 73.66,39.37 73.03,39.37 | 85.72,40.01 87.63,40.01 | 87.63,40.01 97.79,40.01 98.42,39.37 IC13.8 | IC11.8 85.72,40.01 | R6.1 R9.1 R5.1 R8.1 R4.1 R7.1 R3.1 98,18.63 X5.1 | C8.2 87.63,40.01 | R13.1 R14.1 R10.1 R15.2 R19.1 R16.2 R11.1 R17.2 R12.1 R18.2 R20.1 R22.1 R21.1 R23.1 58.63,5.5 58.42,5.71 58.42,8.26 62.23,12.06 X5.26
  Top 0.61: IC4.12 13.34,43.18 | IC3.12 42.55,42.55 | IC2.9 v27.3,38.73 | v27.3,43.81 27.3,42.55 | IC1.9 v56.52,38.73 | v56.52,43.81 56.52,42.55 | 29.61,41.91 C2.2
  Top 0.813: 13.34,43.18 13.97,42.55 27.3,42.55 27.94,42.55 28.57,41.91 29.61,41.91 31.11,41.91 31.75,42.55 42.55,42.55 56.52,42.55 60.33,42.55 | 60.33,42.55 60.33,41.27 61.59,40.01 v61.59,26.04 | 60.33,42.55 60.33,46.48 C1.- 63.37,55.38 X2.2
  Bottom 0.305: v15.24,29.21 15.24,26.04 v13.34,24.13 13.34,17.78 18.41,12.7 18.41,7.62 v19.05,6.99 | v30.48,28.57 v30.48,25.4 | v45.09,29.21 45.72,28.57 v45.72,25.4 | v59.05,26.04 v61.59,26.04
  Bottom 0.406: X5.1 X5.2 92.08,10.16 65.41,10.16 X5.26 X5.25 63.5,24.13 v61.59,26.04
  Bottom 0.813: v27.3,38.73 v27.3,43.81 | v56.52,38.73 v56.52,43.81 | 88.9,60.96 88.9,61.59 87,63.5 64.14,63.5 59.72,59.08 X2.2 | 88.9,60.96 88.9,59.69 X4.2 | J2.1 88.9,60.96
MEN  (via drill 0.6)
  Top 0.305: IC11.7 v84.45,35.56 | v88.9,27.3 88.27,27.3 80.01,19.05 80.01,13.97 78.74,12.7 X5.14 78.74,10.79 80.64,8.89 R10.2
  Bottom 0.305: v84.45,35.56 84.45,31.75 v88.9,27.3
N$1  (via drill 0.6)
  Top 0.305: X4.4 84.45,56.52 v88.27,52.7 | v88.27,33.66 81.92,33.66 80.64,34.92 IC11.4
  Bottom 0.305: v88.27,52.7 v88.27,33.66
N$2  (via drill 0.6)
  Top 0.406: X1.2 38.73,53.34 40.01,52.07 IC3.14 | IC1.12 53.98,51.44 47.62,57.78 v46.35,57.78
  Bottom 0.406: v46.35,57.78 X1.2
N$3  (via drill 0.6)
  Top 0.305: v81.92,53.98 87,48.9 v87,46.99 | v87,34.92 86.36,34.29 83.82,34.29 83.19,34.92 IC11.6
  Bottom 0.305: X4.6 v81.92,53.98 | v87,46.99 v87,34.92
N$4  (via drill 0.6)
  Top 0.406: IC3.16 37.47,50.8 36.2,52.07 v36.2,55.24 X1.4 | IC1.14 51.44,50.16 46.35,55.24 v45.09,55.24
  Bottom 0.406: v45.09,55.24 v36.2,55.24
N$5
  Top 0.305: IC11.10 84.45,49.53 79.38,54.61 X4.8
N$6  (via drill 0.6)
  Top 0.406: IC3.18 34.92,49.53 33.66,50.8 v33.66,52.7 X1.6 | IC1.16 48.9,48.9 45.09,52.7 v43.81,52.7
  Bottom 0.406: v43.81,52.7 v33.66,52.7
N$7
  Top 0.305: IC11.12 81.92,50.8 76.83,55.88 X4.10
N$8  (via drill 0.6)
  Top 0.406: X1.8 v31.11,50.16 31.11,49.53 32.38,48.26 IC3.20 | IC1.18 46.35,47.62 43.81,50.16 v42.55,50.16
  Bottom 0.406: v42.55,50.16 v31.11,50.16
N$9
  Top 0.305: X4.12 74.3,55.88 78.11,52.07 IC11.15
N$10
  Top 0.406: IC3.13 41.27,52.7 40.01,53.98 40.01,59.05 X1.1 46.99,60.33 55.24,52.07 IC1.11
N$11  (via drill 0.6)
  Top 0.305: IC12.2 v65.41,35.56
  Bottom 0.305: v65.41,35.56 65.41,53.98 66.67,55.24 69.22,55.24 X4.14
N$12  (via drill 0.6)
  Top 0.406: X1.3 37.47,59.05 v37.47,56.52 37.47,52.7 38.73,51.44 IC3.15 | IC1.13 52.7,50.8 46.99,56.52 v45.72,56.52
  Bottom 0.406: v45.72,56.52 v37.47,56.52
N$13  (via drill 0.6)
  Top 0.305: X4.16 69.22,53.98 71.75,51.44 71.75,48.9 71.12,48.26 67.31,48.26 v66.67,47.62 | IC12.4 v67.94,35.56
  Bottom 0.305: v67.94,35.56 67.94,46.35 v66.67,47.62
N$14  (via drill 0.6)
  Top 0.406: X1.5 34.92,59.05 v34.92,53.98 34.92,51.44 36.2,50.16 IC3.17 | IC1.15 50.16,49.53 45.72,53.98 v44.45,53.98
  Bottom 0.406: v44.45,53.98 v34.92,53.98
N$15  (via drill 0.6)
  Top 0.305: IC13.6 v95.89,35.56 | v95.89,46.99 85.72,57.15 85.72,59.05 X4.3
  Bottom 0.305: v95.89,35.56 v95.89,46.99
N$16  (via drill 0.6)
  Top 0.406: X1.7 32.38,59.05 v32.38,51.44 32.38,50.16 33.66,48.9 IC3.19 | IC1.17 47.62,48.26 44.45,51.44 v43.18,51.44
  Bottom 0.406: v43.18,51.44 v32.38,51.44
N$17  (via drill 0.6)
  Top 0.305: IC5.4 52.7,30.48 v53.34,31.11 | v55.24,34.29 IC1.8
  Bottom 0.305: v53.34,31.11 54.61,29.84 57.15,29.84 57.78,30.48 57.78,31.75 v55.24,34.29
N$18
  Top 0.305: IC5.2 55.24,32.38 53.98,33.66 IC1.7
N$19
  Top 0.305: IC1.6 52.7,33.66 51.44,32.38 IC5.5
N$20  (via drill 0.6)
  Top 0.305: IC1.5 v51.44,34.29 | v56.52,31.11 IC5.1
  Bottom 0.305: v51.44,34.29 53.34,34.29 v56.52,31.11
N$21  (via drill 0.6)
  Top 0.305: IC1.4 v50.16,33.66 | v51.44,20.95 IC5.12
  Bottom 0.305: v50.16,33.66 50.16,29.21 55.88,23.5 55.88,21.59 56.52,20.95 56.52,19.68 55.88,19.05 52.07,19.05 51.44,19.68 v51.44,20.95
N$22  (via drill 0.6)
  Top 0.305: IC1.3 v48.9,34.29 | v55.24,20.32 IC5.15
  Bottom 0.305: v48.9,34.29 48.9,29.31 IC5.15 v55.24,20.32
N$23  (via drill 0.6)
  Top 0.305: IC1.2 v47.62,33.66 | v53.98,20.95 IC5.14
  Bottom 0.305: v47.62,33.66 47.62,29.31 IC5.14 v53.98,20.95
N$24  (via drill 0.6)
  Top 0.305: IC1.1 v46.35,34.29 | v52.7,20.32 IC5.13
  Bottom 0.305: v46.35,34.29 46.35,29.31 IC5.13 v52.7,20.32
N$25  (via drill 0.6)
  Top 0.305: IC3.5 v37.47,34.29 | v41.27,31.11 IC7.1
  Bottom 0.305: v37.47,34.29 38.1,34.29 v41.27,31.11
N$26
  Top 0.305: IC3.7 IC7.2
N$27  (via drill 0.6)
  Top 0.305: IC7.4 v37.47,31.11 | v41.27,34.29 IC3.8
  Bottom 0.305: v37.47,31.11 39.37,29.21 42.55,29.21 43.18,29.84 43.18,32.38 v41.27,34.29
N$28
  Top 0.305: IC3.6 38.73,33.66 38.1,33.02 37.47,33.02 36.2,31.75 IC7.5
N$29  (via drill 0.6)
  Top 0.305: IC3.4 v36.2,33.66 | v36.2,20.95 IC7.12
  Bottom 0.305: v36.2,33.66 36.2,27.94 40.64,23.5 40.64,21.59 41.27,20.95 41.27,19.68 40.64,19.05 36.83,19.05 36.2,19.68 v36.2,20.95
N$30  (via drill 0.6)
  Top 0.305: IC3.1 v32.38,34.29 | v37.47,20.32 IC7.13
  Bottom 0.305: v32.38,34.29 32.38,28.04 IC7.13 v37.47,20.32
N$31  (via drill 0.6)
  Top 0.305: IC3.2 v33.66,33.66 | v38.73,20.95 IC7.14
  Bottom 0.305: v33.66,33.66 33.66,28.04 IC7.14 v38.73,20.95
N$32  (via drill 0.6)
  Top 0.305: IC3.3 v34.92,34.29 | v40.01,20.32 IC7.15
  Bottom 0.305: v34.92,34.29 34.92,28.04 IC7.15 v40.01,20.32
N$33  (via drill 0.6)
  Top 0.305: IC13.4 v93.34,35.56 | v93.34,46.99 92.08,48.26 90.81,48.26 83.19,55.88 83.19,59.05 X4.5
  Bottom 0.305: v93.34,35.56 v93.34,46.99
N$34  (via drill 0.6)
  Top 0.305: IC13.2 v90.81,35.56 | v90.81,46.99 80.64,57.15 80.64,59.05 X4.7
  Bottom 0.305: v90.81,35.56 v90.81,46.99
N$35  (via drill 0.6)
  Top 0.305: IC8.6 5.71,27.3 6.35,26.67 v16.51,26.67 | IC6.6 20.95,30.48 20.32,31.11 v15.88,31.11 | IC9.10 13.34,11.43 13.97,10.79 17.78,10.79 18.41,11.43 18.41,12.7 19.05,13.34 20.32,13.34 v20.95,12.7
  Bottom 0.305: v15.88,31.11 16.51,30.48 v16.51,26.67 16.51,17.14 v20.95,12.7
N$36
  Top 0.305: C13.1 R1.2 9.53,16.3 IC9.13 IC9.12
N$37  (via drill 0.6)
  Top 0.305: IC12.15 65.41,48.26 66.67,49.53 v70.48,49.53 | v79.38,49.53 79.38,52.07 75.56,55.88 75.56,59.05 X4.9
  Bottom 0.305: v70.48,49.53 v79.38,49.53
N$38  (via drill 0.6)
  Top 0.305: X4.11 73.03,59.05 73.03,55.88 76.83,52.07 v76.83,46.99 | IC12.12 v69.22,46.35
  Bottom 0.305: v69.22,46.35 69.85,46.99 v76.83,46.99
N$39  (via drill 0.6)
  Top 0.305: IC9.6 v14.61,8.89 | IC9.11 v12.06,14.61 13.97,14.61 14.61,13.97 IC9.9
  Bottom 0.305: v12.06,14.61 12.06,11.43 v14.61,8.89
N$40
  Top 0.305: X4.13 70.48,59.05 70.48,53.98 74.3,50.16 74.3,47.62 73.66,46.99 72.39,46.99 71.75,46.35 IC12.10
N$41  (via drill 0.6)
  Top 0.305: X4.15 67.94,59.05 v67.94,53.98 | IC12.6 v70.48,35.56 | v73.03,45.72 73.66,45.72 75.56,47.62 75.56,51.44 v73.03,53.98
  Bottom 0.305: v70.48,35.56 70.48,43.18 v73.03,45.72 | v73.03,53.98 v67.94,53.98
N$42
  Top 0.305: A1.8 123.83,42.76 R24.1 124.04,40.57 Q1.1
N$43  (via drill 0.6)
  Top 0.305: IC5.3 53.98,27.3 53.34,26.67 v29.21,26.67 | IC6.3 v24.77,31.11 | IC10.10 31.11,13.97 v29.84,15.24 | v24.77,3.17 23.5,1.91 18.41,1.91 17.78,2.54 10.79,2.54 9.53,3.81 IC9.2 IC9.1
  Bottom 0.305: v24.77,31.11 24.77,30.48 28.57,26.67 v29.21,26.67 29.21,24.77 29.84,24.13 v29.84,15.24 31.11,13.97 31.11,5.71 32.38,4.45 32.38,3.17 30.48,1.27 26.67,1.27 v24.77,3.17
N$44
  Top 0.305: Q1.3 126.19,38.27 127,37.47 JP2.2
N$45
  Top 0.305: JP2.1 124.46,31.75 123.83,31.11 120.14,31.11 119.38,31.88 JP3.1
N$46  (via drill 0.6)
  Top 0.406: IC2.12 v24.77,49.53 28.57,53.34 X1.10 | IC4.14 10.79,48.26 12.06,49.53 v15.24,49.53
  Bottom 0.406: v15.24,49.53 v24.77,49.53
N$48  (via drill 0.6)
  Top 0.406: IC2.14 22.23,50.8 v23.5,52.07 26.04,54.61 X1.12 | IC4.16 8.26,48.26 12.06,52.07 v13.97,52.07
  Bottom 0.406: v13.97,52.07 v23.5,52.07
N$50  (via drill 0.6)
  Top 0.406: IC2.16 19.68,52.07 v22.23,54.61 23.5,55.88 X1.14 | IC4.18 5.71,48.26 12.06,54.61 v12.7,54.61
  Bottom 0.406: v12.7,54.61 v22.23,54.61
N$52
  Top 0.406: IC2.18 17.14,53.98 X1.16 12.06,57.78 3.17,48.9 IC4.20
N$54  (via drill 0.6)
  Top 0.406: IC2.11 v26.04,48.26 26.04,48.9 29.84,52.7 29.84,59.05 X1.9 | IC4.13 12.06,47.62 12.7,48.26 v15.88,48.26
  Bottom 0.406: v15.88,48.26 v26.04,48.26
N$56  (via drill 0.6)
  Top 0.406: IC2.13 23.5,50.16 v24.13,50.8 27.3,53.98 27.3,59.05 X1.11 | IC4.15 9.53,48.26 12.06,50.8 v14.61,50.8
  Bottom 0.406: v14.61,50.8 v24.13,50.8
N$58  (via drill 0.6)
  Top 0.406: IC2.15 20.95,51.44 v22.86,53.34 24.77,55.24 24.77,59.05 X1.13 | IC4.17 6.99,48.26 12.06,53.34 v13.34,53.34
  Bottom 0.406: v13.34,53.34 v22.86,53.34
N$60  (via drill 0.6)
  Top 0.406: IC2.17 18.41,52.7 v21.59,55.88 22.23,56.52 22.23,59.05 X1.15 | IC4.19 4.45,48.26 v12.06,55.88
  Bottom 0.406: v12.06,55.88 v21.59,55.88
N$61  (via drill 0.6)
  Top 0.305: IC6.4 v23.5,31.75 | v26.04,34.29 IC2.8
  Bottom 0.305: v23.5,31.75 24.13,32.38 25.4,32.38 26.04,31.75 26.04,30.48 26.67,29.84 27.94,29.84 28.57,30.48 28.57,31.75 v26.04,34.29
N$62
  Top 0.305: IC2.7 24.77,33.66 26.04,32.38 IC6.2
N$63
  Top 0.305: IC2.6 23.5,33.66 22.23,32.38 IC6.5
N$64  (via drill 0.6)
  Top 0.305: IC6.1 v27.3,31.11 | v22.23,34.29 IC2.5
  Bottom 0.305: v27.3,31.11 27.3,31.75 26.04,33.02 25.4,33.02 24.13,34.29 v22.23,34.29
N$65  (via drill 0.6)
  Top 0.305: IC2.4 v20.95,33.66 | v22.23,20.95 IC6.12
  Bottom 0.305: v20.95,33.66 20.95,29.21 27.3,22.86 27.3,19.68 26.67,19.05 22.86,19.05 22.23,19.68 v22.23,20.95
N$66  (via drill 0.6)
  Top 0.305: IC2.3 v19.68,34.29 | v26.04,20.32 IC6.15
  Bottom 0.305: v19.68,34.29 19.68,29.31 IC6.15 v26.04,20.32
N$67  (via drill 0.6)
  Top 0.305: IC2.2 v18.41,33.66 | v24.77,20.95 IC6.14
  Bottom 0.305: v18.41,33.66 18.41,29.21 24.77,22.86 v24.77,20.95
N$68  (via drill 0.6)
  Top 0.305: IC2.1 v17.14,34.29 | v23.5,20.32 IC6.13
  Bottom 0.305: v17.14,34.29 17.14,29.31 IC6.13 v23.5,20.32
N$69  (via drill 0.6)
  Top 0.305: IC8.1 v12.06,31.11 | v8.26,34.29 IC4.5
  Bottom 0.305: v12.06,31.11 10.16,33.02 9.53,33.02 v8.26,34.29
N$70
  Top 0.305: IC4.7 IC8.2
N$71  (via drill 0.6)
  Top 0.305: IC8.4 8.26,30.48 v8.89,31.11 | v12.06,34.29 IC4.8
  Bottom 0.305: v8.89,31.11 10.16,29.84 12.7,29.84 13.34,30.48 13.34,33.02 v12.06,34.29
N$72
  Top 0.305: IC4.6 9.53,33.66 6.99,31.11 IC8.5
N$73  (via drill 0.6)
  Top 0.305: IC4.4 v6.99,33.66 | v6.99,20.95 IC8.12
  Bottom 0.305: v6.99,33.66 6.99,31.11 10.16,27.94 10.16,23.5 12.06,21.59 12.06,19.68 11.43,19.05 7.62,19.05 6.99,19.68 v6.99,20.95
N$74  (via drill 0.6)
  Top 0.305: IC8.13 v8.26,20.32 | v3.17,34.29 IC4.1
  Bottom 0.305: v8.26,20.32 8.26,26.04 3.17,31.11 v3.17,34.29
N$75  (via drill 0.6)
  Top 0.305: IC4.2 v4.45,33.66 | v9.53,20.95 IC8.14
  Bottom 0.305: v4.45,33.66 4.45,31.11 8.89,26.67 8.89,21.59 v9.53,20.95
N$76  (via drill 0.6)
  Top 0.305: IC8.15 v10.79,20.32 | v5.71,34.29 IC4.3
  Bottom 0.305: v10.79,20.32 10.79,21.59 9.53,22.86 9.53,27.3 5.71,31.11 v5.71,34.29
N$77  (via drill 0.6)
  Top 0.305: IC5.6 50.16,27.94 49.53,27.3 43.81,27.3 | 43.81,27.3 35.56,27.3 34.92,27.94 IC7.6 | 43.81,27.3 v43.81,28.57 | v18.41,4.45 17.78,3.81 12.7,3.81 12.06,4.45 IC9.4 | v43.81,16.51 43.18,17.14 36.2,17.14 34.29,15.24 31.75,15.24 29.84,17.14 22.86,17.14 v21.59,15.88
  Bottom 0.305: v43.81,28.57 v43.81,16.51 | v21.59,15.88 22.23,15.24 22.23,8.26 v18.41,4.45
N$100
  Top 0.305: IC9.5 13.34,5.08 13.97,4.45 15.88,4.45 17.14,5.71 19.68,5.71 20.32,5.08 20.32,3.81 20.95,3.17 22.86,3.17 24.77,5.08 IC10.2
N$101  (via drill 0.6)
  Top 0.305: C13.2 13.97,16.51 15.88,14.61 22.23,14.61 22.86,15.24 26.67,15.24 v27.3,15.88 | v27.3,4.45 IC10.4
  Bottom 0.305: v27.3,15.88 v27.3,4.45
N$102  (via drill 0.6)
  Top 0.305: IC8.10 4.45,19.68 5.71,18.41 19.05,18.41 v19.68,17.78 20.32,18.41 33.02,18.41 v33.66,17.78 34.29,18.41 48.26,18.41 v48.9,17.78 | IC5.10 v48.9,20.32 | IC7.10 v33.66,20.95 | IC6.10 v19.68,20.95 | IC10.6 v29.84,4.45
  Bottom 0.305: v48.9,20.32 v48.9,17.78 | v33.66,20.95 v33.66,17.78 | v19.68,20.95 v19.68,17.78 20.32,18.41 27.3,18.41 28.57,17.14 28.57,14.61 29.84,13.34 v29.84,4.45
N$104
  Top 0.305: IC9.8 15.88,13.97 22.86,13.97 23.5,14.61 27.94,14.61 28.57,13.97 IC10.12
N$105  (via drill 0.6)
  Top 0.305: IC8.9 3.17,19.68 5.08,17.78 17.78,17.78 v18.41,17.14 19.05,16.51 20.32,16.51 21.59,17.78 31.11,17.78 v32.38,16.51 34.29,16.51 35.56,17.78 46.35,17.78 v47.62,16.51 | IC5.9 v47.62,20.95 | IC7.9 v32.38,20.32 | IC6.9 v18.41,20.32 | IC10.15 v24.77,10.16
  Bottom 0.305: v47.62,20.95 v47.62,16.51 | v32.38,20.32 v32.38,16.51 | v18.41,20.32 v18.41,17.14 19.05,16.51 20.32,16.51 20.95,17.14 22.86,17.14 24.77,15.24 v24.77,10.16
N$106  (via drill 0.6)
  Top 0.305: IC8.11 5.71,19.68 6.35,19.05 20.95,19.05 | 20.95,19.05 34.92,19.05 | 34.92,19.05 49.53,19.05 v50.16,19.68 IC5.11 | IC6.11 20.95,19.05 | IC7.11 34.92,19.05 | IC11.2 78.11,26.67 v74.93,23.5 | v64.77,23.5 63.5,23.5 v58.42,18.41
  Bottom 0.305: v50.16,19.68 51.44,18.41 v58.42,18.41 | v74.93,23.5 v64.77,23.5
N$110  (via drill 0.6)
  Top 0.305: IC8.3 9.53,27.94 10.16,27.3 13.97,27.3 | 13.97,27.3 15.24,27.3 15.88,27.94 17.14,27.94 17.78,27.3 27.94,27.3 29.21,28.57 29.21,29.21 31.11,31.11 v31.11,33.66 | 13.97,27.3 v13.97,28.57 | v19.05,3.17 11.43,3.17 10.79,3.81 IC9.3 | IC7.3 v38.73,31.75
  Bottom 0.305: v13.97,28.57 12.06,26.67 12.06,23.5 12.7,22.86 12.7,17.14 17.78,12.06 17.78,6.35 16.51,5.08 16.51,3.81 17.14,3.17 v19.05,3.17 | v31.11,33.66 31.11,34.92 31.75,35.56 38.1,35.56 41.27,32.38 41.91,32.38 42.55,31.75 42.55,30.48 41.91,29.84 40.64,29.84 v38.73,31.75
RA0  (via drill 0.6)
  Top 0.305: X5.7 86.36,20.32 v87.63,21.59 95.89,29.84 R9.2 | IC11.3 79.38,34.92 81.92,32.38 v81.92,27.94
  Bottom 0.305: v81.92,27.94 81.92,27.3 v87.63,21.59
RA1
  Top 0.305: IC10.7 31.11,5.71 33.02,3.81 85.72,3.81 86.36,4.45 X5.8 86.36,12.7 87.63,13.97 87.63,19.68 95.89,27.94 R5.2
RA2  (via drill 0.6)
  Top 0.305: v31.11,3.81 31.75,3.17 86.36,3.17 87.63,4.45 87.63,12.7 88.9,13.97 X5.5 88.9,19.68 95.25,26.04 R8.2 | IC10.14 v26.04,10.79
  Bottom 0.305: v26.04,10.79 26.04,3.17 27.3,1.91 29.21,1.91 v31.11,3.81
RD  (via drill 0.6)
  Top 0.305: 32.38,12.7 IC10.9 32.38,11.43 v33.66,10.16 | v33.66,5.08 34.29,4.45 85.09,4.45 85.72,5.08 85.72,10.16 X5.10 85.09,13.34 85.09,21.59 88.27,24.77 89.53,24.77 91.44,26.67 91.44,27.94 95.25,31.75 R6.2
  Bottom 0.305: v33.66,5.08 v33.66,10.16
REN0
  Top 0.305: IC10.3 26.04,3.17 27.94,1.27 88.27,1.27 91.44,4.45 X5.4 91.44,12.7 92.71,13.97 92.71,19.05 93.98,20.32 R3.2
REN1  (via drill 0.6)
  Top 0.305: v27.94,3.17 29.21,1.91 87.63,1.91 90.17,4.45 90.17,12.7 91.44,13.97 X5.3 91.44,19.68 93.98,22.23 R7.2 | v28.57,10.16 29.21,10.16 29.84,10.79 IC10.11
  Bottom 0.305: v27.94,3.17 28.57,3.81 v28.57,10.16
SEL1  (via drill 0.6)
  Top 0.305: v71.75,31.11 71.75,24.13 73.66,22.23 X5.17 73.66,13.97 72.39,12.7 72.39,10.79 71.12,9.53 R17.1 | v66.67,45.72 IC12.14
  Bottom 0.305: v71.75,31.11 70.48,31.11 66.67,34.92 v66.67,45.72
SEL2  (via drill 0.6)
  Top 0.305: IC12.11 v70.48,45.72 | v70.48,33.66 70.48,23.5 71.12,22.86 X5.19 71.12,13.97 69.85,12.7 69.85,10.79 67.31,8.26 R18.1
  Bottom 0.305: v70.48,45.72 69.22,44.45 69.22,34.92 v70.48,33.66
SEL3  (via drill 0.6)
  Top 0.305: v68.58,24.77 X5.21 68.58,13.97 67.31,12.7 67.31,11.43 63.5,7.62 R22.2 | v73.03,24.77 v73.03,35.56 | v74.3,43.81 73.13,43.81 IC12.9
  Bottom 0.305: v68.58,24.77 v73.03,24.77 | v73.03,35.56 73.03,42.55 v74.3,43.81
SEL4
  Top 0.305: IC12.3 66.67,28.57 69.85,25.4 69.85,13.97 68.58,12.7 X5.22 68.58,11.43 65.41,8.26 R20.2
SEL5  (via drill 0.6)
  Top 0.305: v65.41,29.84 66.04,29.21 X5.23 66.04,13.97 64.77,12.7 64.77,11.43 62.87,9.53 60.96,9.53 59.69,8.26 R23.2 | v71.75,33.02 IC12.7
  Bottom 0.305: v65.41,29.84 72.39,29.84 73.03,30.48 73.03,31.75 v71.75,33.02
SEL6  (via drill 0.6)
  Top 0.305: IC12.5 v69.22,27.94 | v67.31,26.04 67.31,13.97 66.04,12.7 X5.24 66.04,11.43 63.5,8.89 62.23,8.89 61.81,8.47 61.81,7.2 R21.2
  Bottom 0.305: v69.22,27.94 v67.31,26.04
VCC
  Top 0.305: IC14.3 109.22,26.67 108.58,27.3 106.05,27.3 105.41,26.67 105.41,25.4 104.78,24.77 103.5,24.77 102.87,25.4 102.87,29.21 103.11,29.45 C9.1 106.28,29.45 106.68,29.84 IC14.16 106.68,40.64 103.5,43.81 103.5,48.26 113.67,58.42 A1.27
VIN
  Bottom 0.61: A1.30 104.14,62.87 J1.2

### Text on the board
tPlace: + 12VDC - | ROWS | COLUMN DRIVER | GND | Flip dot master | Flip dot row driver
